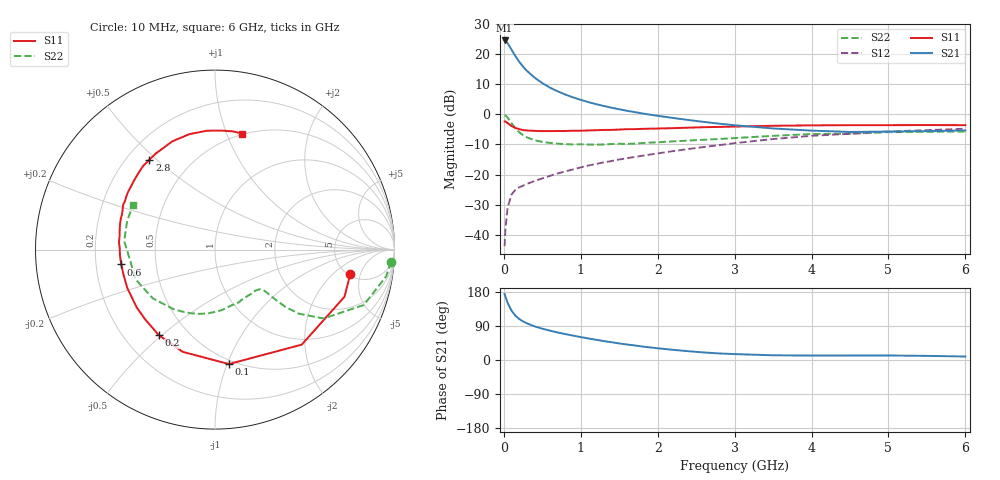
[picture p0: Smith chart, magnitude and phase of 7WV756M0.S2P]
! Infineon Technologies  Discrete & RF Semiconductors
! BFS17W
! Si NPN RF Bipolar Junction Transistor in SOT323
! VCE = 0.75 V  IC = 6 mA
! Common Emitter S-Parameters:  August  1999
# GHz  S  MA  R  50
!  f  S11  S21  S12  S22
! GHz  MAG  ANG  MAG  ANG  MAG  ANG  MAG  ANG
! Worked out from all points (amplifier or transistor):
!   36 points, 10 MHz to 6 GHz, reference 50 ohm
!   highest |S21| = 24.7 dB at 10 MHz (marker M1)
!   |S21| within 3 dB of that: start of sweep to 98.02 MHz
!   unconditionally stable (mu >= 1): 439 MHz to end of sweep
!   at 250 MHz: K = 0.70, MSG = 19.8 dB, |S12| = -23.7 dB
!   at 1.4 GHz: K = 1.36, MAG = 5.3 dB, |S12| = -15.5 dB
!   at 6 GHz: K = 1.13, MAG = -2.5 dB, |S12| = -4.8 dB
!   S11 on the Smith chart (normalised r, x): 10 MHz: 5.26, -3.42; 100 MHz: 0.47, -1.01; 200 MHz: 0.35, -0.49; 600 MHz: 0.31, -0.07; 2.8 GHz: 0.29, +0.47; 6 GHz: 0.49, +1.14
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0.01  0.7659 -10.1  17.11 174.3  0.0064 83.8  0.9835 -4.0
0.02  0.7678 -20.0  16.93 167.6  0.0125 81.7  0.9653 -8.9
0.05  0.7169 -47.6  15.34 150.5  0.0284 68.9  0.8848 -20.4
0.1  0.6424 -83.1  12 130.2  0.0467 53.4  0.7164 -32.4
0.15  0.5973 -107.5  9.384 116.8  0.0555 46.6  0.5874 -37.4
0.2  0.5702 -123.3  7.561 108.2  0.0612 44.7  0.5063 -39.1
0.25  0.5501 -135.1  6.269 101.7  0.0653 43.1  0.4502 -39.5
0.3  0.5422 -143.6  5.337 96.7  0.0698 43.5  0.4157 -39.7
0.4  0.5335 -156.3  4.105 88.7  0.078 45.1  0.3715 -39.7
0.5  0.5287 -164.6  3.331 82.7  0.0862 47.6  0.3496 -39.9
0.6  0.5287 -171.0  2.799 77.4  0.0949 49.3  0.336 -41.0
0.8  0.531 179.2  2.149 68.3  0.113 52.2  0.3207 -45.7
0.9  0.5366 175.6  1.924 64.4  0.1217 53.1  0.3171 -48.2
1.1  0.5422 168.3  1.606 56.7  0.1413 54.2  0.3159 -54.5
1.3  0.5525 161.8  1.385 49.9  0.1594 54.7  0.3163 -61.9
1.6  0.5696 154.0  1.152 40.9  0.1867 55.2  0.3235 -72.8
2.2  0.5923 139.8  0.875 26.8  0.2453 54.6  0.3564 -95.6
2.8  0.6203 126.1  0.703 17.3  0.3088 51.8  0.3909 -118.0
3.5  0.6483 111.5  0.585 12.4  0.3903 46.1  0.4405 -142.0
4.5  0.6638 93.9  0.512 11.8  0.478 34.6  0.4784 -173.9
5.5  0.6661 81.5  0.527 10.9  0.5488 24.1  0.5147 162.0
6  0.6638 76.7  0.544 9.2  0.5777 19.1  0.5208 151.4
